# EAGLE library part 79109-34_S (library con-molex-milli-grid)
RECEPTACAL
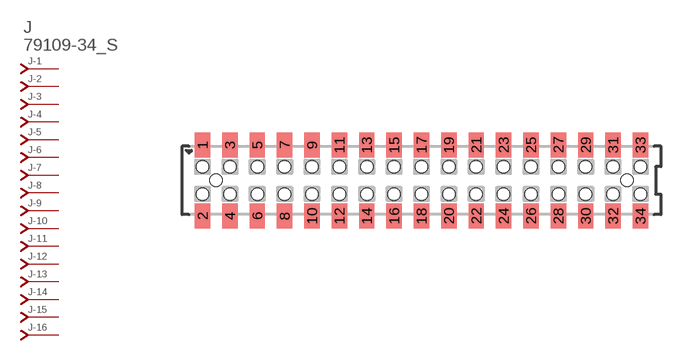
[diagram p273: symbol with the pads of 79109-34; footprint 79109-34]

Designator prefix J; gates -1=J-NV -2=J-N -3=J-N -4=J-N -5=J-N -6=J-N -7=J-N -8=J-N -9=J-N -10=J-N -11=J-N -12=J-N -13=J-N -14=J-N -15=J-N -16=J-N -17=J-N -18=J-N -19=J-N -20=J-N -21=J-N -22=J-N -23=J-N -24=J-N -25=J-N -26=J-N -27=J-N -28=J-N -29=J-N -30=J-N -31=J-N -32=J-N -33=J-N -34=J-N

## 79109-34_S  [79109-34]
1  -1:J  pas
2  -2:J  pas
3  -3:J  pas
4  -4:J  pas
5  -5:J  pas
6  -6:J  pas
7  -7:J  pas
8  -8:J  pas
9  -9:J  pas
10  -10:J  pas
11  -11:J  pas
12  -12:J  pas
13  -13:J  pas
14  -14:J  pas
15  -15:J  pas
16  -16:J  pas
17  -17:J  pas
18  -18:J  pas
19  -19:J  pas
20  -20:J  pas
21  -21:J  pas
22  -22:J  pas
23  -23:J  pas
24  -24:J  pas
25  -25:J  pas
26  -26:J  pas
27  -27:J  pas
28  -28:J  pas
29  -29:J  pas
30  -30:J  pas
31  -31:J  pas
32  -32:J  pas
33  -33:J  pas
34  -34:J  pas

## Footprint 79109-34 (pad centres in mm)
RECEPTACAL SMD Dual Row, Vertical, Pass-Thru
smd 1.12 x 1.83: 1 -16,2.6; 2 -16,-2.6; 3 -14,2.6; 4 -14,-2.6; 5 -12,2.6; 6 -12,-2.6; 7 -10,2.6; 8 -10,-2.6; 9 -8,2.6; 10 -8,-2.6; 11 -6,2.6; 12 -6,-2.6; 13 -4,2.6; 14 -4,-2.6; 15 -2,2.6; 16 -2,-2.6; 17 0,2.6; 18 0,-2.6; 19 2,2.6; 20 2,-2.6; 21 4,2.6; 22 4,-2.6; 23 6,2.6; 24 6,-2.6; 25 8,2.6; 26 8,-2.6; 27 10,2.6; 28 10,-2.6; 29 12,2.6; 30 12,-2.6; 31 14,2.6; 32 14,-2.6; 33 16,2.6; 34 16,-2.6
hole 0.914 at -15,0
hole 0.914 at -16,1
hole 0.914 at -16,-1
hole 0.914 at -14,-1
hole 0.914 at -14,1
hole 0.914 at -12,-1
hole 0.914 at -12,1
hole 0.914 at 15,0
hole 0.914 at -10,1
hole 0.914 at -10,-1
hole 0.914 at -8,1
hole 0.914 at -8,-1
hole 0.914 at -6,1
hole 0.914 at -6,-1
hole 0.914 at -4,1
hole 0.914 at -4,-1
hole 0.914 at -2,-1
hole 0.914 at -2,1
hole 0.914 at 0,1
hole 0.914 at 0,-1
hole 0.914 at 2,1
hole 0.914 at 2,-1
hole 0.914 at 4,1
hole 0.914 at 4,-1
hole 0.914 at 6,-1
hole 0.914 at 6,1
hole 0.914 at 8,1
hole 0.914 at 10,1
hole 0.914 at 12,1
hole 0.914 at 8,-1
hole 0.914 at 10,-1
hole 0.914 at 12,-1
hole 0.914 at 14,-1
hole 0.914 at 16,-1
hole 0.914 at 14,1
hole 0.914 at 16,1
